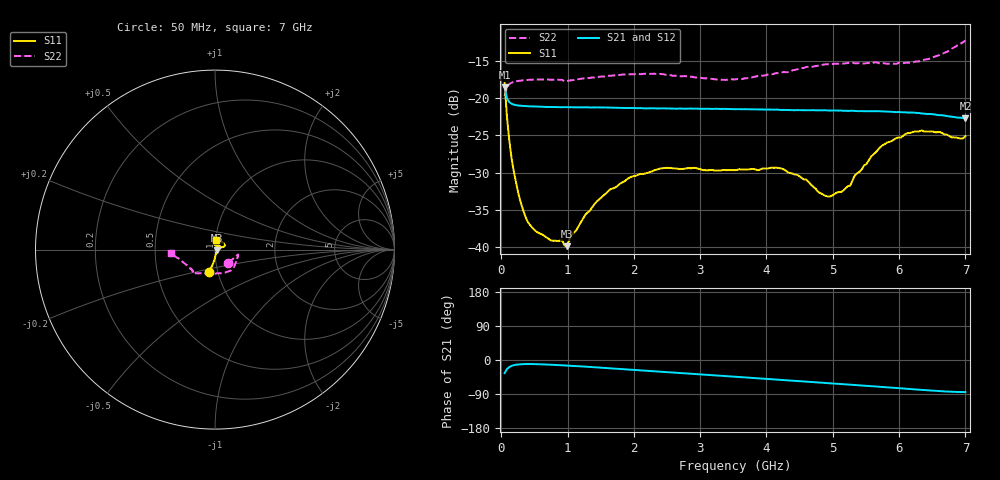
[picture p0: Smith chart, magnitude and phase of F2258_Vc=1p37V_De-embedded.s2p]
! Integrated Device Technology
! Corporate Headquarters
! 6024 Silver Creek Valley Road
! San Jose, CA 95138  USA
! Phone:  1-408-284-8200
! Toll Free:  1-800-223-1366
! Webpage:  http://www.idt.com/
! Timing and RF Division
! 515 Groton Road, Suite 102
! Westford, MA 01886-6024
! Device:  F2258
! Description: Voltage Variable RF Attenuator
! Frequency:  50.0 -  6000.00 MHz
! Package:  3x3 mm Thin QFN Plastic Package: 16 pin
! Ports:  2 RF, 2 DC
!  Pin  1  = NC
!  Pin  2  = NC
!  Pin  3  = RF2  = Port 2
!  Pin  4  = GND
!  Pin  5  = Vdd
!  Pin  6  = NC
!  Pin  7  = VCTRL
!  Pin  8  = NC
!  Pin  9  = GND
!  Pin 10  = RF1  = Port 1
!  Pin 11  = NC
!  Pin 12  = NC
!  Pin 13  = NC
!  Pin 14  = NC
!  Pin 15  = NC
!  Pin 16  = NC
! Vcntrl:  1.370 Volts
! Vdd:  +3.300 Volts
! Current:  1.166 mA
! Data:  The device was measured on a the F2258 evaluation board which has
!  individual transmission lines to the RF pins.  Data was collected
!  using a calibrated network analyzer.  The evaluation board was
!  de-embedded using a TRL calibration technique.
!  The reference plane is the edge of the package pin.
! Misc:  SN 10
!  Action Tracker AT0285
! Date Measured:  2014-12-10
! Date:  2016-01-13  MJV
! Note:
!  Integrated Device Technology supplies this data as a sample of measured
!  data at the package pin for this product.  Your particular data for this
!  product may vary.
!  Data was taken at 25 degrees C.
!  Integrated Device Technology reserves the right to change this data at anytime.
!Freq_(GHz)  S11M_(dB)  S11P_(deg)  S21M_(dB)  S21P_(deg)  S12M_(dB)  S12P_(deg)  S22M_(dB)  S22P_(deg)
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# GHz S dB R 50
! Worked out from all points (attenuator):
!   201 points, 50 MHz to 7 GHz, reference 50 ohm
!   highest |S21| = -18.49 dB at 50 MHz (marker M1); lowest = -22.7 dB at 7 GHz (marker M2)
!   lowest |S11| = -39.9 dB at 988.2 MHz (marker M3), VSWR 1.02, Z = 50.9 - j0.42 ohm
!   |S11| at or under -10 dB: start of sweep to end of sweep
!   |S22| runs from -19.7 to -12.2 dB; largest |S21 - S12| = 0.00076
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0.05  -17.96 -104.6  -18.49 -34.6  -18.54 -34.7  -19.70 -44.5
0.08475  -22.42 -97.2  -19.98 -24.1  -20.04 -24.2  -18.58 -22.0
0.15425  -28.02 -88.7  -20.73 -15.6  -20.78 -15.6  -17.90 -13.8
0.2585  -32.82 -77.5  -20.98 -11.7  -21.00 -11.7  -17.66 -11.9
0.36275  -35.89 -65.7  -21.06 -10.7  -21.07 -10.7  -17.56 -12.8
0.5365  -37.98 -46.4  -21.11 -11.0  -21.13 -11.0  -17.47 -15.5
0.98825  -39.88 -24.0  -21.20 -14.6  -21.20 -14.6  -17.69 -26.1
1.05775  -38.33 -16.3  -21.21 -15.3  -21.22 -15.3  -17.58 -27.5
1.2315  -36.17 -5.8  -21.22 -17.1  -21.22 -17.1  -17.34 -31.2
1.6485  -32.22 5.1  -21.26 -21.9  -21.26 -21.9  -16.97 -39.8
2.37825  -29.49 25.3  -21.36 -30.3  -21.37 -30.3  -16.73 -54.7
3.525  -29.67 78.6  -21.47 -44.1  -21.48 -44.0  -17.46 -92.0
4.22  -29.42 101.1  -21.58 -52.5  -21.56 -52.5  -16.57 -116.5
4.7065  -31.89 89.2  -21.59 -58.4  -21.58 -58.4  -15.74 -126.1
4.915  -33.18 69.6  -21.64 -61.0  -21.60 -61.1  -15.42 -128.4
5.1235  -32.59 48.5  -21.64 -63.5  -21.61 -63.5  -15.37 -130.6
5.2625  -31.73 34.2  -21.69 -65.1  -21.66 -65.2  -15.20 -131.9
5.332  -30.36 28.4  -21.69 -66.1  -21.66 -66.2  -15.30 -132.0
5.57525  -27.86 19.1  -21.73 -69.0  -21.70 -69.1  -15.30 -135.1
5.85325  -25.87 17.8  -21.81 -72.6  -21.77 -72.7  -15.34 -139.1
6.33975  -24.32 26.3  -22.05 -79.0  -22.01 -79.1  -14.95 -151.3
7  -25.09 83.7  -22.67 -84.7  -22.63 -84.9  -12.23 -175.0
